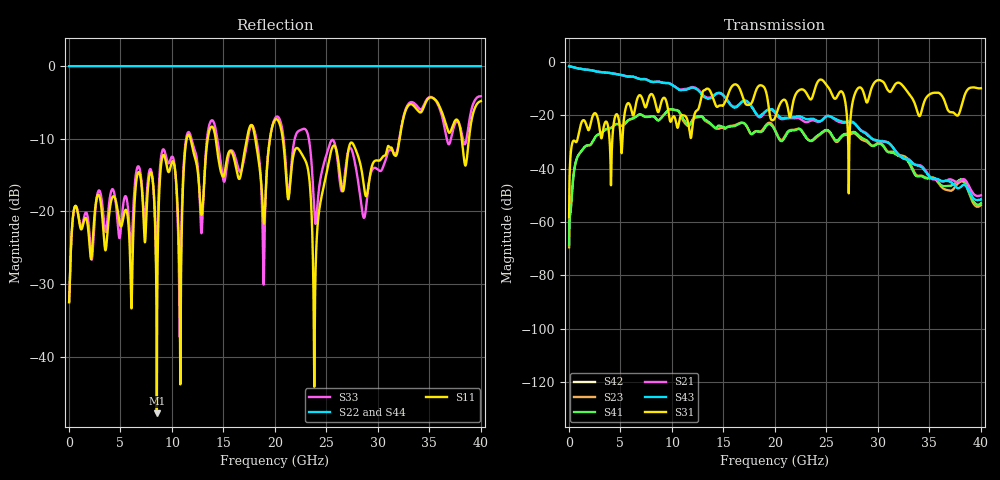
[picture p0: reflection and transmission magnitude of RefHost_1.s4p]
# GHz S RI R 50
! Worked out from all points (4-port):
!   4000 points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, 10 MHz to 40 GHz, reference 50 ohm
!   strongest paths, dB at 10 MHz, 10.01 GHz, 20.01 GHz, 30.01 GHz, 40 GHz:
!     S31: -58.2, -21.3, -20.9, -6.9, -9.9
!     S43: -1.6, -8.7, -18.7, -29.6, -51.5
!     S21: -1.6, -8.6, -19.2, -29.7, -50.0
!     S41: -68.7, -17.8, -25.9, -30.7, -53.0
!     S23: -69.4, -17.9, -25.5, -30.3, -53.6
!     S42: -, -, -, -, -
!   lowest |S11| = -47.8 dB at 8.53 GHz (marker M1), VSWR 1.01, Z = 49.8 + j0.374 ohm
!   |S11| at or under -10 dB: start of sweep to 11.43 GHz; 14.25 GHz to 17.28 GHz (3.031 GHz wide, 19.2 % of centre); 20.76 GHz to 32.1 GHz (11.34 GHz wide, 42.9 % of centre)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
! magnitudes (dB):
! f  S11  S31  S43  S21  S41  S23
! 10 MHz  -32.5  -58.2  -1.6  -1.6  -68.7  -69.4
! 1.37 GHz  -21.8  -21.9  -2.8  -2.8  -32.6  -32.6
! 8.53 GHz  -47.8  -17.8  -7.5  -7.4  -21.6  -21.6
! 11.6 GHz  -9.5  -23.4  -10.2  -9.9  -23.5  -24.1
! 20.27 GHz  -7.4  -17.9  -20.0  -20.5  -28.1  -27.7
! 23.85 GHz  -38.0  -10.5  -21.6  -22.1  -28.5  -28.9
! 40 GHz  -4.8  -9.9  -51.5  -50.0  -53.0  -53.6
